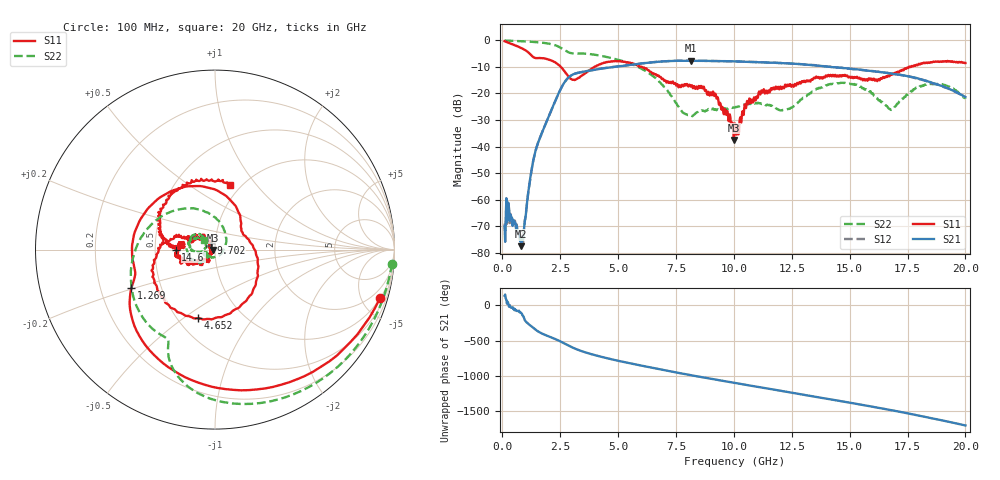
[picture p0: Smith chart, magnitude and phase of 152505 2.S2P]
!  2-Port S-parameters saved by WinCal
! VAR MeasName=S-Parameters (CALIBRATED_DATA) read from VNA (N5230C)
! VAR MeasDate=4/10/2015 9:28:38 AM
! VAR NAME=152505 2
! VAR FILENAME=152505 2.S2P
! VAR DATE=4/10/2015 9:28:38 AM
! VAR PHYS_PORTS=1,2
# Hz S DB R 50
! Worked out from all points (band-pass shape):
!   801 points, 100 MHz to 20 GHz, reference 50 ohm
!   highest |S21| = -7.70 dB at 8.135 GHz (marker M1); lowest = -77.5 dB at 821.4 MHz (marker M2)
!   |S21| within 3 dB of the highest: 4.265 GHz to 15 GHz (10.73 GHz wide, 111 % of centre)
!   lowest |S11| = -37.5 dB at 10 GHz (marker M3), VSWR 1.03, Z = 48.7 - j0.2 ohm
!   |S11| at or under -10 dB: 2.523 GHz to 3.974 GHz (1.451 GHz wide, 44.7 % of centre); 5.951 GHz to 5.998 GHz (46.7 MHz wide, 0.782 % of centre); 6.023 GHz to 17.58 GHz (11.55 GHz wide, 97.9 % of centre)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
!   |S22| runs from -28.6 to -0.1 dB; largest |S21 - S12| = 0.0067
!   S11 on the Smith chart (normalised r, x): 100 MHz: 1.03, -6.80; 1.269 GHz: 0.34, -0.20; 4.652 GHz: 0.63, -0.57; 9.702 GHz: 0.95, +0.08; 14.6 GHz: 0.64, +0.00; 20 GHz: 0.89, +0.75
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1e8  -0.37 -16.4  -70.15 137.9  -69.03 163.5  -0.08 -4.6
2.74125e8  -0.92 -41.0  -61.80 -4.8  -61.82 -5.2  -0.17 -11.5
8.21375e8  -2.94 -108.8  -77.50 -110.0  -74.68 -121.6  -0.38 -33.3
1.269125e9  -5.79 -155.3  -48.67 60.4  -48.65 61.3  -0.59 -51.4
2.289e9  -8.34 112.9  -22.79 -117.5  -22.79 -117.5  -1.89 -97.0
2.861125e9  -13.64 45.4  -14.03 149.7  -14.02 149.9  -4.56 -116.2
3.43325e9  -13.40 3.6  -11.97 69.9  -11.96 70.3  -5.00 -126.7
4.652125e9  -8.09 -104.2  -10.25 -39.8  -10.21 -39.6  -6.58 -170.9
5.62225e9  -8.63 -162.0  -9.18 -109.0  -9.14 -109.3  -9.10 148.0
6.741625e9  -13.22 158.9  -8.10 177.5  -8.08 177.1  -15.21 87.6
8.134625e9  -17.43 156.0  -7.70 90.2  -7.73 90.1  -28.46 -66.6
9.179375e9  -20.61 128.9  -7.83 29.0  -7.81 28.9  -25.97 -139.1
9.70175e9  -26.79 120.4  -7.89 -1.0  -7.88 -1.0  -25.68 -144.1
1.000025e10  -37.54 -171.1  -7.93 -18.2  -7.95 -18.0  -25.30 -141.6
1.005e10  -31.33 -156.7  -7.94 -21.1  -7.96 -21.1  -25.28 -140.7
1.119425e10  -18.89 -136.3  -8.29 -85.6  -8.26 -86.0  -24.01 -159.6
1.231362e10  -16.76 -150.9  -8.69 -148.5  -8.69 -149.1  -25.95 -145.6
1.338325e10  -14.82 -157.7  -9.39 150.4  -9.33 150.5  -19.29 -137.8
1.460212e10  -13.21 179.9  -10.40 81.9  -10.31 81.0  -16.07 -179.6
1.669162e10  -13.52 179.7  -12.39 -40.9  -12.42 -42.0  -25.71 158.5
1.843288e10  -8.44 138.6  -15.61 -154.8  -15.84 -155.5  -16.36 165.9
2e10  -8.59 76.7  -21.37 95.5  -21.46 95.9  -22.07 139.2
